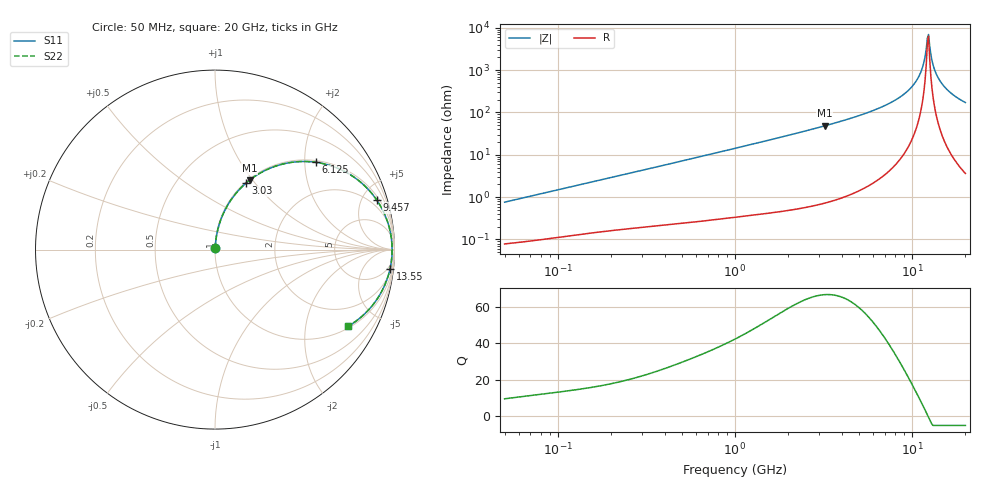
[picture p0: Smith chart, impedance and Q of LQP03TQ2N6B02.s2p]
!Murata Part Number: LQP03TQ2N6B02
!These Parameters are Measured in Series Mode Connection
!  o--[Z]--o
!Port1  Port2
!  o-------o
!Freq. Start=50[MHz] Stop=20[GHz], 401[Steps]
# Hz S RI R 50
!Freq.(Hz) S11(Real) S11(Imag) S21(Real) S21(Imag) S12(Real) S12(Imag) S22(Real) S22(Imag)
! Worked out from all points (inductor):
!   401 points, 50 MHz to 20 GHz, reference 50 ohm
!   read as one part in series: L = 2.39 nH near 51.52 MHz
!   highest Q = 66.8 at 3.217 GHz (marker M1), where L = 2.39 nH
!   self-resonance near 12.2 GHz
!   S11 on the Smith chart (normalised r, x): 50 MHz: 1.00, +0.02; 3.03 GHz: 1.01, +0.90; 6.125 GHz: 1.04, +2.27; 9.457 GHz: 1.29, +6.41; 13.55 GHz: 3, -18; 20 GHz: 1.07, -3.41
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5e7  0.000843 0.00756  0.9992 -0.00756  0.9992 -0.00756  0.000843 0.00756
1.364002e8  0.00173 0.0199  0.9983 -0.0199  0.9983 -0.0199  0.00173 0.0199
3.721004e8  0.00491 0.0528  0.9951 -0.0528  0.9951 -0.0528  0.00491 0.0528
1e9  0.0228 0.138  0.9772 -0.138  0.9772 -0.138  0.0228 0.138
2.728004e9  0.1423 0.3418  0.8577 -0.3418  0.8577 -0.3418  0.1423 0.3418
3.029571e9  0.1725 0.3704  0.8275 -0.3704  0.8275 -0.3704  0.1725 0.3704
3.216634e9  0.1924 0.3868  0.8076 -0.3868  0.8076 -0.3868  0.1924 0.3868
4.472136e9  0.3433 0.467  0.6567 -0.467  0.6567 -0.467  0.3433 0.467
6.125241e9  0.5621 0.4864  0.4379 -0.4864  0.4379 -0.4864  0.5621 0.4864
7.442007e9  0.7227 0.4351  0.2773 -0.4351  0.2773 -0.4351  0.7227 0.4351
9.457416e9  0.9011 0.2766  0.0989 -0.2766  0.0989 -0.2766  0.9011 0.2766
1.034674e10  0.9479 0.1909  0.0521 -0.1909  0.0521 -0.1909  0.9479 0.1909
1.115139e10  0.9738 0.1117  0.0262 -0.1117  0.0262 -0.1117  0.9738 0.1117
1.149051e10  0.9804 0.0787  0.0196 -0.0787  0.0196 -0.0787  0.9804 0.0787
1.201863e10  0.986 0.0282  0.014 -0.0282  0.014 -0.0282  0.986 0.0282
1.220001e10  0.9867 0.0113  0.0133 -0.0113  0.0133 -0.0113  0.9867 0.0113
1.257102e10  0.9864 -0.0226  0.0136 0.0226  0.0136 0.0226  0.9864 -0.0226
1.314879e10  0.9816 -0.0732  0.0184 0.0732  0.0184 0.0732  0.9816 -0.0732
1.354865e10  0.9755 -0.1064  0.0245 0.1064  0.0245 0.1064  0.9755 -0.1064
1.438523e10  0.9568 -0.1707  0.0432 0.1707  0.0432 0.1707  0.9568 -0.1707
1.573793e10  0.9138 -0.2593  0.0862 0.2593  0.0862 0.2593  0.9138 -0.2593
2e10  0.7402 -0.428  0.2598 0.428  0.2598 0.428  0.7402 -0.428
